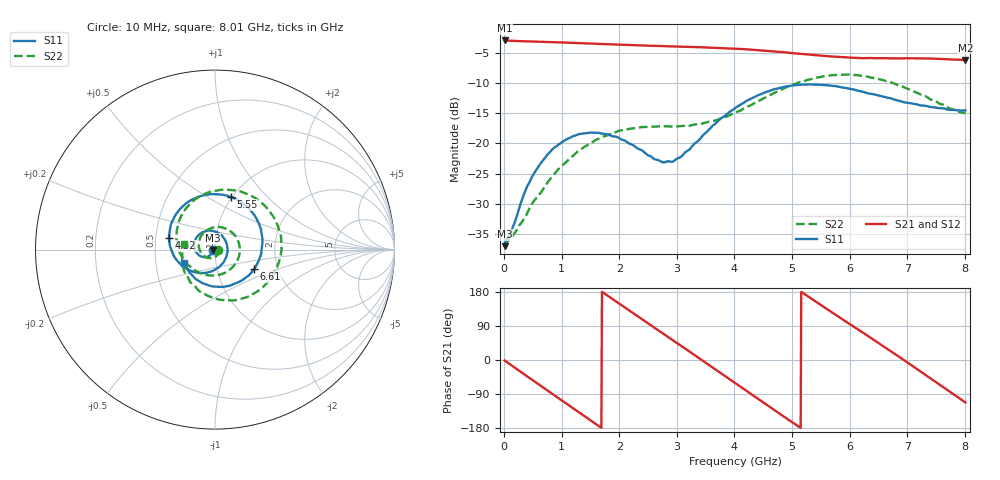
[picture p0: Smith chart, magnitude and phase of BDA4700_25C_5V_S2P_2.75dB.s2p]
!Agilent Technologies,E5071B,MY42404982,A.09.10
!Date: Mon Oct 20 13:27:16 2025
!Data & Calibration Information:
!Freq	S11:SOLT2(ON)	S21:SOLT2(ON)	S12:SOLT2(ON)	S22:SOLT2(ON)
# Hz S RI R 50
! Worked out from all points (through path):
!   801 points, 10 MHz to 8.01 GHz, reference 50 ohm
!   highest |S21| = -2.86 dB at 10 MHz (marker M1); lowest = -6.1 dB at 8.01 GHz (marker M2)
!   group delay of S21, straight-line fit = 288 ps
!   lowest |S11| = -37.1 dB at 10 MHz (marker M3), VSWR 1.03, Z = 48.6 - j0.17 ohm
!   |S11| at or under -10 dB: start of sweep to end of sweep
!   |S22| runs from -36.4 to -8.5 dB; largest |S21 - S12| = 0.0056
!   S11 on the Smith chart (normalised r, x): 10 MHz: 0.97, -0.00; 4.52 GHz: 0.59, +0.08; 5.55 GHz: 0.98, +0.64; 6.61 GHz: 1.51, -0.34; 8.01 GHz: 0.70, -0.11
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1e7  -0.0139 -0.00174  0.7189 -0.0155  0.719 -0.0165  0.0162 -0.00159
3.3e8  -0.0235 -0.0274  0.5765 -0.4118  0.5761 -0.4127  0.0178 -0.0144
7.1e8  -0.0632 -0.0419  0.1712 -0.6778  0.1708 -0.6783  -0.00453 -0.0438
1.02e9  -0.1018 -0.0195  -0.2201 -0.6553  -0.2203 -0.6557  -0.0514 -0.0418
1.35e9  -0.1161 0.0323  -0.5469 -0.4078  -0.5476 -0.4081  -0.0896 0.0125
1.64e9  -0.0935 0.0794  -0.6698 -0.0738  -0.6702 -0.0736  -0.0739 0.0805
1.93e9  -0.0451 0.1047  -0.6074 0.2709  -0.6076 0.271  -0.00633 0.1236
2.32e9  0.026 0.0869  -0.2816 0.5909  -0.2814 0.5915  0.1014 0.0896
2.68e9  0.066 0.03  0.1325 0.6331  0.1323 0.6331  0.1377 -0.0152
3.36e9  0.0134 -0.1032  0.6269 0.0835  0.6274 0.0829  -0.00293 -0.144
3.67e9  -0.0662 -0.1303  0.5671 -0.2617  0.567 -0.2632  -0.0906 -0.1261
4.01e9  -0.1685 -0.1009  0.3038 -0.5351  0.3039 -0.5348  -0.1676 -0.0646
4.52e9  -0.2562 0.0662  -0.2406 -0.541  -0.2411 -0.5416  -0.2121 0.11
4.95e9  -0.1826 0.2379  -0.5297 -0.2058  -0.53 -0.2077  -0.1131 0.2777
5.35e9  -0.0107 0.3089  -0.5138 0.1842  -0.5145 0.1832  0.0954 0.331
5.55e9  0.0864 0.2935  -0.4107 0.3434  -0.411 0.3433  0.208 0.2962
6.07e9  0.2537 0.1211  0.0191 0.5152  0.0191 0.5171  0.3697 0.0414
6.61e9  0.219 -0.1068  0.4261 0.2843  0.426 0.2836  0.2417 -0.2295
6.68e9  0.2007 -0.1305  0.4569 0.2289  0.4577 0.2284  0.208 -0.2496
7.23e9  0.0143 -0.2068  0.4416 -0.2557  0.4419 -0.2568  -0.0529 -0.2506
7.62e9  -0.1052 -0.1656  0.1636 -0.4764  0.1624 -0.477  -0.1689 -0.1254
8.01e9  -0.1732 -0.0741  -0.1867 -0.4583  -0.1863 -0.4592  -0.1755 0.0324
